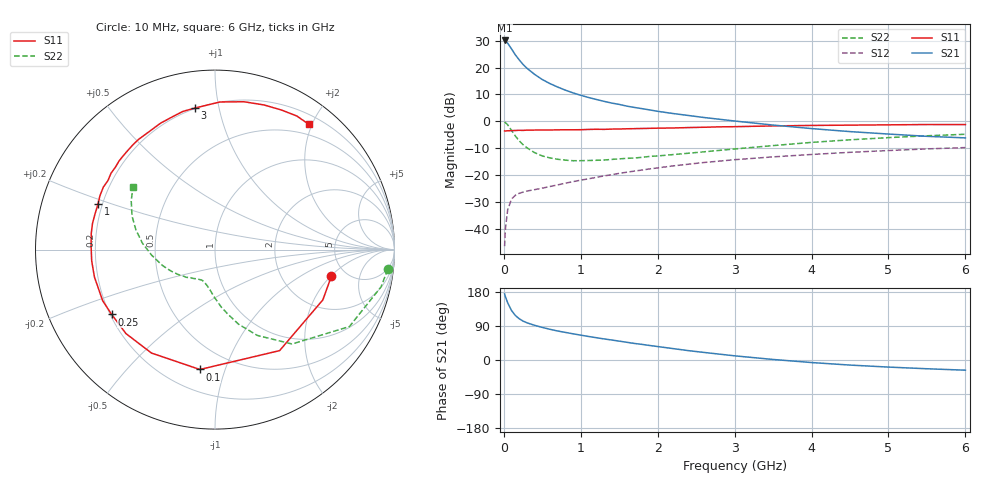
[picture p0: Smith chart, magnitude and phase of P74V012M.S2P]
! SIEMENS Small Signal Semiconductors
! BFP196
! Si NPN RF Bipolar Junction Transistor in SOT143
! VCE = 4 V  IC = 12 mA
! Common Emitter S-Parameters:  May  1996
# GHz  S  MA  R  50
!  f  S11  S21  S12  S22
! GHz  MAG  ANG  MAG  ANG  MAG  ANG  MAG  ANG
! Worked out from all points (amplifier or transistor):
!   36 points, 10 MHz to 6 GHz, reference 50 ohm
!   highest |S21| = 30.1 dB at 10 MHz (marker M1)
!   |S21| within 3 dB of that: start of sweep to 96.41 MHz
!   unconditionally stable (mu >= 1): 841.1 MHz to 3.346 GHz
!   at 250 MHz: K = 0.45, MSG = 23.7 dB, |S12| = -26.3 dB
!   at 1.4 GHz: K = 1.13, MAG = 11.2 dB, |S12| = -19.8 dB
!   at 6 GHz: K = 0.96, MSG = 1.8 dB, |S12| = -9.7 dB
!   S11 on the Smith chart (normalised r, x): 10 MHz: 3.83, -2.04; 100 MHz: 0.34, -0.82; 250 MHz: 0.21, -0.28; 1 GHz: 0.18, +0.18; 3 GHz: 0.20, +0.85; 6 GHz: 0.34, +1.96
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0.01  0.6652 -12.9  31.83 174.4  0.0048 86.2  0.9688 -6.5
0.02  0.663 -25.0  31.13 167.2  0.01 78.9  0.9485 -12.6
0.05  0.6681 -57.4  28.28 150.9  0.0227 64.7  0.8629 -29.8
0.1  0.6733 -97.2  22.14 130.6  0.0361 49.2  0.6787 -50.8
0.15  0.6764 -121.6  17.17 117.4  0.0424 41.4  0.5327 -63.8
0.2  0.682 -136.7  13.87 108.9  0.0461 37.4  0.4357 -72.5
0.25  0.6796 -147.9  11.39 102.7  0.0485 35.4  0.3672 -78.7
0.3  0.6876 -155.5  9.704 98.2  0.0507 35.3  0.3228 -83.7
0.4  0.6889 -167.2  7.458 91.5  0.0539 35.7  0.2621 -91.3
0.5  0.6898 -174.8  5.979 86.0  0.0574 37.4  0.2278 -96.7
0.6  0.6907 178.3  5.027 81.0  0.0617 39.1  0.2092 -101.2
0.7  0.6953 172.5  4.336 76.5  0.066 40.7  0.1974 -105.4
0.8  0.6979 168.0  3.798 72.8  0.071 41.8  0.1903 -109.1
1  0.6994 158.7  3.047 65.6  0.0808 44.3  0.1858 -114.5
1.1  0.7078 155.0  2.778 62.1  0.0857 45.1  0.1875 -117.0
1.6  0.7276 137.3  1.916 46.7  0.1137 46.0  0.2053 -129.7
2.2  0.753 119.0  1.398 30.1  0.1487 42.9  0.2413 -143.6
3  0.7964 98.2  1.015 11.0  0.194 35.3  0.3069 -163.5
3.5  0.8229 88.1  0.853 1.4  0.2188 29.9  0.3545 -175.0
4.5  0.8509 71.3  0.645 -13.4  0.266 18.9  0.4542 166.0
5.5  0.8729 58.5  0.527 -23.1  0.3076 7.8  0.5394 149.9
6  0.8721 53.1  0.493 -26.9  0.3258 1.7  0.576 142.6
